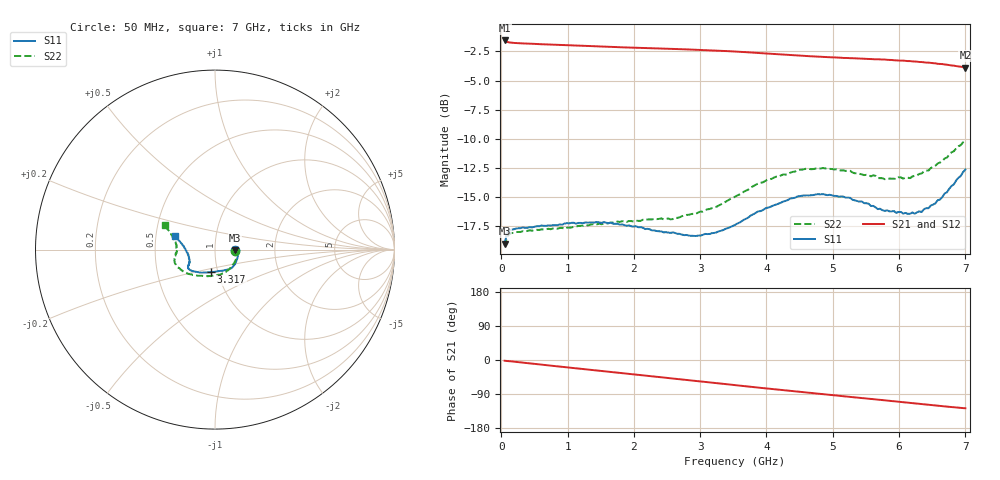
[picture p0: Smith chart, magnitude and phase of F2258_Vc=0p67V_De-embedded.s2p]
! Integrated Device Technology
! Corporate Headquarters
! 6024 Silver Creek Valley Road
! San Jose, CA 95138  USA
! Phone:  1-408-284-8200
! Toll Free:  1-800-223-1366
! Webpage:  http://www.idt.com/
! Timing and RF Division
! 515 Groton Road, Suite 102
! Westford, MA 01886-6024
! Device:  F2258
! Description: Voltage Variable RF Attenuator
! Frequency:  50.0 -  6000.00 MHz
! Package:  3x3 mm Thin QFN Plastic Package: 16 pin
! Ports:  2 RF, 2 DC
!  Pin  1  = NC
!  Pin  2  = NC
!  Pin  3  = RF2  = Port 2
!  Pin  4  = GND
!  Pin  5  = Vdd
!  Pin  6  = NC
!  Pin  7  = VCTRL
!  Pin  8  = NC
!  Pin  9  = GND
!  Pin 10  = RF1  = Port 1
!  Pin 11  = NC
!  Pin 12  = NC
!  Pin 13  = NC
!  Pin 14  = NC
!  Pin 15  = NC
!  Pin 16  = NC
! Vcntrl:  0.670 Volts
! Vdd:  +3.300 Volts
! Current:  1.114 mA
! Data:  The device was measured on a the F2258 evaluation board which has
!  individual transmission lines to the RF pins.  Data was collected
!  using a calibrated network analyzer.  The evaluation board was
!  de-embedded using a TRL calibration technique.
!  The reference plane is the edge of the package pin.
! Misc:  SN 10
!  Action Tracker AT0285
! Date Measured:  2014-12-10
! Date:  2016-01-13  MJV
! Note:
!  Integrated Device Technology supplies this data as a sample of measured
!  data at the package pin for this product.  Your particular data for this
!  product may vary.
!  Data was taken at 25 degrees C.
!  Integrated Device Technology reserves the right to change this data at anytime.
!Freq_(GHz)  S11M_(dB)  S11P_(deg)  S21M_(dB)  S21P_(deg)  S12M_(dB)  S12P_(deg)  S22M_(dB)  S22P_(deg)
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# GHz S dB R 50
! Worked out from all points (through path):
!   201 points, 50 MHz to 7 GHz, reference 50 ohm
!   highest |S21| = -1.55 dB at 50 MHz (marker M1); lowest = -3.9 dB at 7 GHz (marker M2)
!   group delay of S21, straight-line fit = 50.5 ps
!   lowest |S11| = -19.0 dB at 50 MHz (marker M3), VSWR 1.25, Z = 62.6 - j0.516 ohm
!   |S11| at or under -10 dB: start of sweep to end of sweep
!   |S22| runs from -19.2 to -10.1 dB; largest |S21 - S12| = 0.0012
!   S11 on the Smith chart (normalised r, x): 50 MHz: 1.25, -0.01; 3.317 GHz: 0.93, -0.24; 7 GHz: 0.63, +0.10
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0.05  -19.02 -2.1  -1.55 -2.0  -1.55 -2.0  -19.23 -2.6
0.08475  -18.17 -3.4  -1.67 -2.5  -1.67 -2.5  -18.43 -4.1
0.15425  -17.80 -5.5  -1.74 -3.7  -1.74 -3.7  -18.10 -7.2
0.71025  -17.44 -23.9  -1.89 -14.2  -1.88 -14.2  -17.74 -30.2
1.2315  -17.25 -39.9  -2.01 -23.9  -2.00 -23.9  -17.47 -51.2
1.6485  -17.21 -49.1  -2.10 -31.5  -2.10 -31.5  -17.20 -64.0
2.37825  -17.95 -64.0  -2.24 -44.8  -2.25 -44.8  -16.89 -83.6
2.58675  -18.05 -69.8  -2.28 -48.7  -2.28 -48.7  -16.90 -90.2
2.93425  -18.36 -82.5  -2.35 -55.1  -2.35 -55.1  -16.46 -102.6
3.3165  -17.91 -99.7  -2.44 -62.3  -2.44 -62.3  -15.63 -118.0
3.525  -17.40 -109.3  -2.50 -66.3  -2.50 -66.3  -14.99 -126.2
4.0115  -15.93 -128.3  -2.68 -75.3  -2.67 -75.3  -13.53 -143.1
4.46325  -14.97 -139.5  -2.84 -83.5  -2.84 -83.5  -12.72 -155.2
4.7065  -14.84 -142.9  -2.92 -87.8  -2.92 -87.8  -12.61 -159.8
5.2625  -15.08 -148.9  -3.08 -97.4  -3.08 -97.4  -12.76 -168.8
5.5405  -15.59 -151.3  -3.15 -102.2  -3.14 -102.2  -13.13 -173.4
5.6795  -16.05 -153.1  -3.17 -104.5  -3.16 -104.5  -13.38 -175.1
5.85325  -16.24 -157.0  -3.23 -107.6  -3.22 -107.7  -13.43 -179.8
6.166  -16.45 -165.2  -3.33 -113.2  -3.32 -113.2  -13.39 173.6
6.33975  -16.30 -172.8  -3.41 -116.3  -3.41 -116.3  -12.98 169.0
6.61775  -15.22 174.1  -3.57 -121.1  -3.57 -121.1  -12.04 162.0
7  -12.65 161.1  -3.88 -127.4  -3.88 -127.4  -10.11 153.9
